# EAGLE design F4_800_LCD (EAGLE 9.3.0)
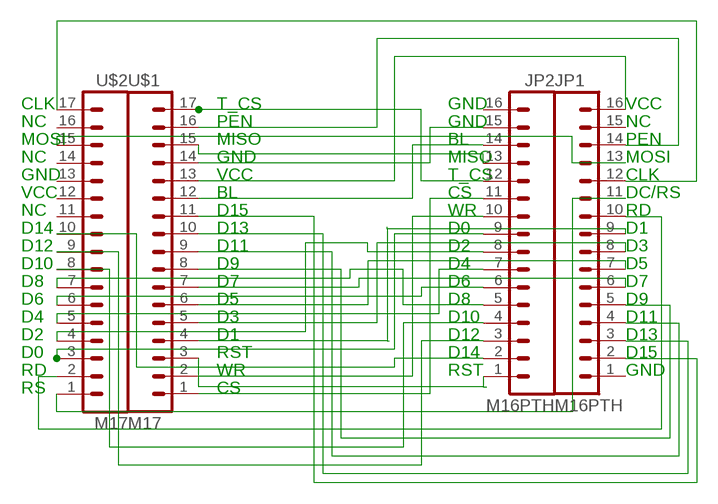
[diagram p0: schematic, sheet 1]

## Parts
JP1  M16PTH  [1X16]
JP2  M16PTH  [1X16]
U$1  M17  [1X17]
U$2  M17  [1X17]

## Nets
N$1: JP2.15 U$1.14
N$2: JP2.14 U$1.12
N$3: JP2.13 U$1.15
N$4: JP1.13 U$2.15
N$5: JP2.12 U$1.17
N$6: JP2.11 U$1.1
N$7: JP2.10 U$1.2
N$8: JP2.1 U$1.3
N$9: JP1.11 U$2.1
N$10: JP1.10 U$2.2
N$11: JP1.16 U$1.13
N$12: JP1.14 U$1.16
N$13: JP2.8 U$2.4
N$14: JP1.12 U$2.17
N$15: JP2.9 U$2.3
N$17: JP1.9 U$1.4
N$19: JP1.8 U$1.5
N$20: JP2.7 U$2.5
N$21: JP1.7 U$1.6
N$22: JP2.6 U$2.6
N$23: JP1.6 U$1.7
N$24: JP2.5 U$2.7
N$25: JP1.5 U$1.8
N$26: JP2.4 U$2.8
N$27: JP1.4 U$1.9
N$28: JP2.3 U$2.9
N$29: JP1.3 U$1.10
N$30: JP2.2 U$2.10
N$31: JP1.2 U$1.11
Unconnected: JP1.1 JP1.15 JP2.16 U$2.11 U$2.12 U$2.13 U$2.14 U$2.16

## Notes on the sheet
- CLK | T_CS | GND | VCC
- NC | PEN | GND | NC
- MOSI | MISO | BL | PEN
- NC | GND | MISO | MOSI
- GND | VCC | T_CS | CLK
- VCC | BL | CS | DC/RS
- NC | D15 | WR | RD
- D14 | D13 | D0 | D1
- D12 | D11 | D2 | D3
- D10 | D9 | D4 | D5
- D8 | D7 | D6 | D7
- D6 | D5 | D8 | D9
- D4 | D3 | D10 | D11
- D2 | D1 | D12 | D13
- D0 | RST | D14 | D15
- RD | WR | RST | GND
- RS | CS

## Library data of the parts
JP1 JP2 = 98 SparkFun:M16
U$1 U$2 = 98 SparkFun:M17

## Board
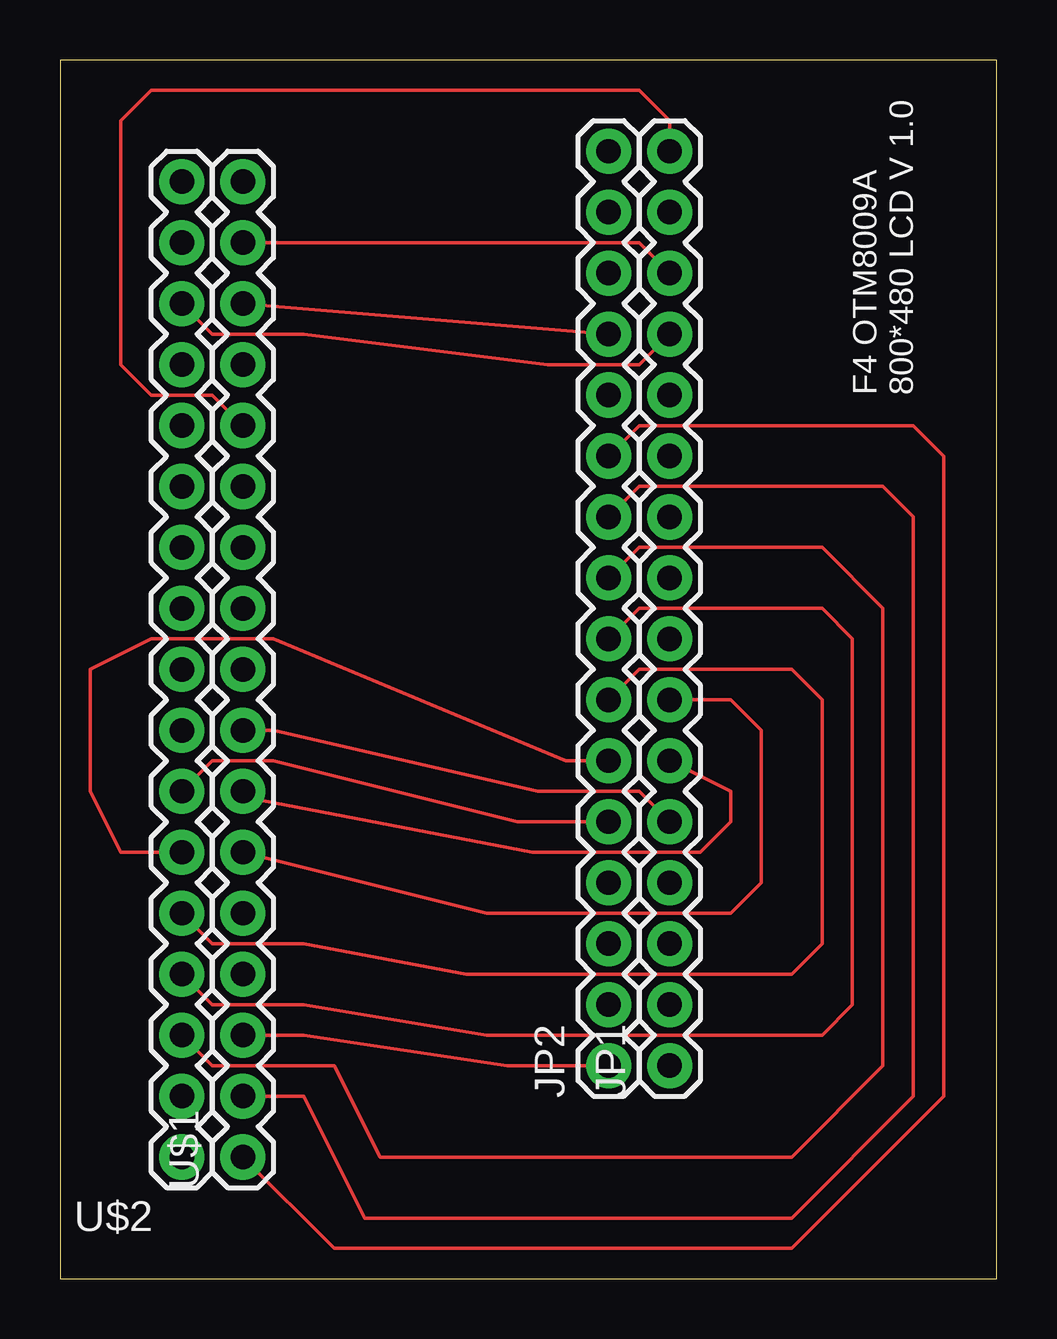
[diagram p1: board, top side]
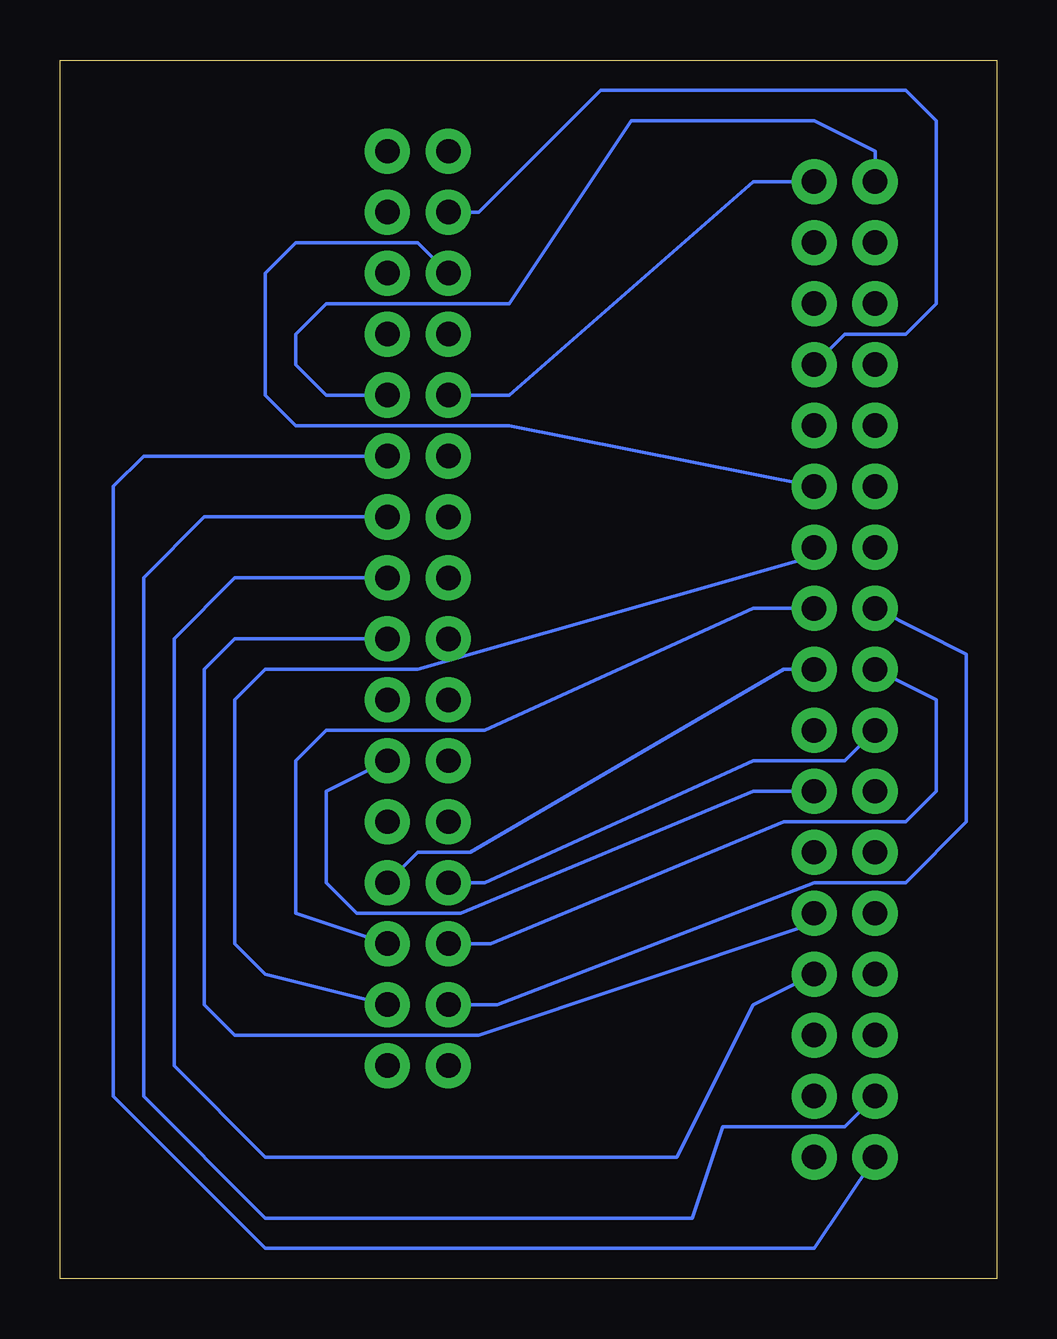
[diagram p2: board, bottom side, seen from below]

Size 39.04 x 50.79 mm. Coordinates in mm from the lower left corner, seen from the top.
Outline: 0,0 39.04,0 39.04,50.79 0,50.79 0,0
Copper layers (1*16): Top 0.035mm / dielectric 1.5mm / Bottom 0.035mm
Design rules "default": minimum track width 6mil, minimum drill 0.35mm, track to track 6mil, track to pad 6mil, pad to pad 6mil, via to via 6mil, smd to smd 6mil, copper to edge 40mil, drill to drill 6mil, minimum pad ring 10mil, minimum via ring 8mil, stop-mask expansion 4mil, vias tented up to drill 0mil, thermal gap 10mil

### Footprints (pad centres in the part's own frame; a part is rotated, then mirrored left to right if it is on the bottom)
1X16 = drill 1.016 pad 1.88: 1 0,0; 2 2.54,0; 3 5.08,0; 4 7.62,0; 5 10.16,0; 6 12.7,0; 7 15.24,0; 8 17.78,0; 9 20.32,0; 10 22.86,0; 11 25.4,0; 12 27.94,0; 13 30.48,0; 14 33.02,0; 15 35.56,0; 16 38.1,0
1X17 = drill 1.016 pad 1.88: 1 0,0; 2 2.54,0; 3 5.08,0; 4 7.62,0; 5 10.16,0; 6 12.7,0; 7 15.24,0; 8 17.78,0; 9 20.32,0; 10 22.86,0; 11 25.4,0; 12 27.94,0; 13 30.48,0; 14 33.02,0; 15 35.56,0; 16 38.1,0; 17 40.64,0

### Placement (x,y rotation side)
JP1  25.4,8.89 90 top
JP2  22.86,8.89 90 top
U$1  7.62,5.08 90 top
U$2  5.08,5.08 90 top

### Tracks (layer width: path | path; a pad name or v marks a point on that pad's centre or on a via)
N$1
  Bottom 0.152: JP2.15 21.59,44.45 16.51,49.53 3.81,49.53 2.54,48.26 2.54,40.64 3.81,39.37 6.35,39.37 U$1.14
N$2
  Bottom 0.152: JP2.14 24.13,43.18 29.21,43.18 30.48,41.91 30.48,36.83 29.21,35.56 20.32,35.56 U$1.12
N$3
  Top 0.152: JP2.13 U$1.15
N$4
  Top 0.152: JP1.13 24.13,38.1 20.32,38.1 10.16,39.37 6.35,39.37 U$2.15
N$5
  Bottom 0.152: JP2.12 20.32,36.83 10.16,45.72 U$1.17
N$6
  Top 0.152: JP2.11 24.13,35.56 35.56,35.56 36.83,34.29 36.83,7.62 30.48,1.27 11.43,1.27 U$1.1
N$7
  Top 0.152: 8.89,7.62 U$1.2 10.16,7.62 12.7,2.54 30.48,2.54 35.56,7.62 35.56,31.75 34.29,33.02 24.13,33.02 JP2.10
N$8
  Top 0.152: JP2.1 18.63,8.89 10.16,10.16 U$1.3
N$9
  Bottom 0.152: JP1.11 35.56,34.29 36.83,33.02 36.83,7.62 30.48,1.27 7.62,1.27 U$2.1
N$10
  Bottom 0.152: JP1.10 33.02,31.75 35.56,29.21 35.56,7.62 30.48,2.54 12.7,2.54 11.43,6.35 6.35,6.35 U$2.2
N$11
  Top 0.152: JP1.16 25.4,48.26 24.13,49.53 3.81,49.53 2.54,48.26 2.54,38.1 3.81,36.83 6.35,36.83 U$1.13
N$12
  Top 0.152: JP1.14 24.13,43.18 U$1.16
N$13
  Top 0.152: JP2.8 24.13,27.94 31.75,27.94 33.02,26.67 33.02,11.43 31.75,10.16 17.78,10.16 10.16,11.43 6.35,11.43 U$2.4
N$14
  Bottom 0.152: U$2.17 5.08,46.99 7.62,48.26 15.24,48.26 20.32,40.64 24.13,40.64 27.94,40.64 29.21,39.37 29.21,38.1 27.94,36.83 JP1.12
N$15
  Top 0.152: JP2.9 24.13,30.48 31.75,30.48 34.29,27.94 34.29,8.89 30.48,5.08 13.34,5.08 11.43,8.89 6.35,8.89 U$2.3
N$17
  Bottom 0.152: JP1.9 31.75,29.21 34.29,26.67 34.29,8.89 30.48,5.08 13.34,5.08 10.16,11.43 U$1.4
N$19
  Bottom 0.152: JP1.8 31.75,26.67 33.02,25.4 33.02,11.43 31.75,10.16 21.59,10.16 8.26,14.61 U$1.5
N$20
  Top 0.152: JP2.7 24.13,25.4 30.48,25.4 31.75,24.13 31.75,13.97 30.48,12.7 16.93,12.7 10.16,13.97 6.35,13.97 U$2.5
N$21
  Top 0.152: JP1.7 27.94,24.13 29.21,22.86 29.21,16.51 27.94,15.24 17.78,15.24 U$1.6
N$22
  Top 0.152: U$2.6 2.54,17.78 1.27,20.32 1.27,25.4 3.81,26.67 8.89,26.67 21.08,21.59 JP2.6
N$23
  Top 0.152: JP1.6 27.94,20.32 27.94,19.05 26.67,17.78 19.68,17.78 7.92,20.02 U$1.7
  Bottom 0.152: JP1.6 27.94,20.32 27.94,16.51 26.67,15.24 22.35,15.24 10.16,20.32 U$1.7
N$24
  Top 0.152: 22.34,19.57 JP2.5 19.05,19.05 8.89,21.59 6.35,21.59 U$2.7
N$25
  Top 0.152: JP1.5 24.13,20.32 19.9,20.32 8.89,22.86 U$1.8
N$26
  Bottom 0.152: U$2.8 6.35,21.59 10.16,21.59 21.34,16.51 JP2.4
N$27
  Bottom 0.152: JP1.4 24.13,17.78 21.95,17.78 8.89,25.4 U$1.9
N$28
  Bottom 0.152: U$2.9 2.54,24.13 2.54,20.32 3.81,19.05 8.89,19.05 21.08,13.97 JP2.3
N$29
  Bottom 0.152: JP1.3 29.21,15.24 29.21,21.59 27.94,22.86 21.34,22.86 10.16,27.94 U$1.10
N$30
  Bottom 0.152: U$2.10 1.27,26.04 1.27,19.05 3.81,16.51 7.62,16.51 20.83,11.43 JP2.2
N$31
  Bottom 0.152: JP1.2 30.48,12.7 31.75,13.97 31.75,24.13 30.48,25.4 24.13,25.4 8.13,29.97 U$1.11

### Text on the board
_tsilk: F4 OTM8009A / 800*480 LCD V 1.0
